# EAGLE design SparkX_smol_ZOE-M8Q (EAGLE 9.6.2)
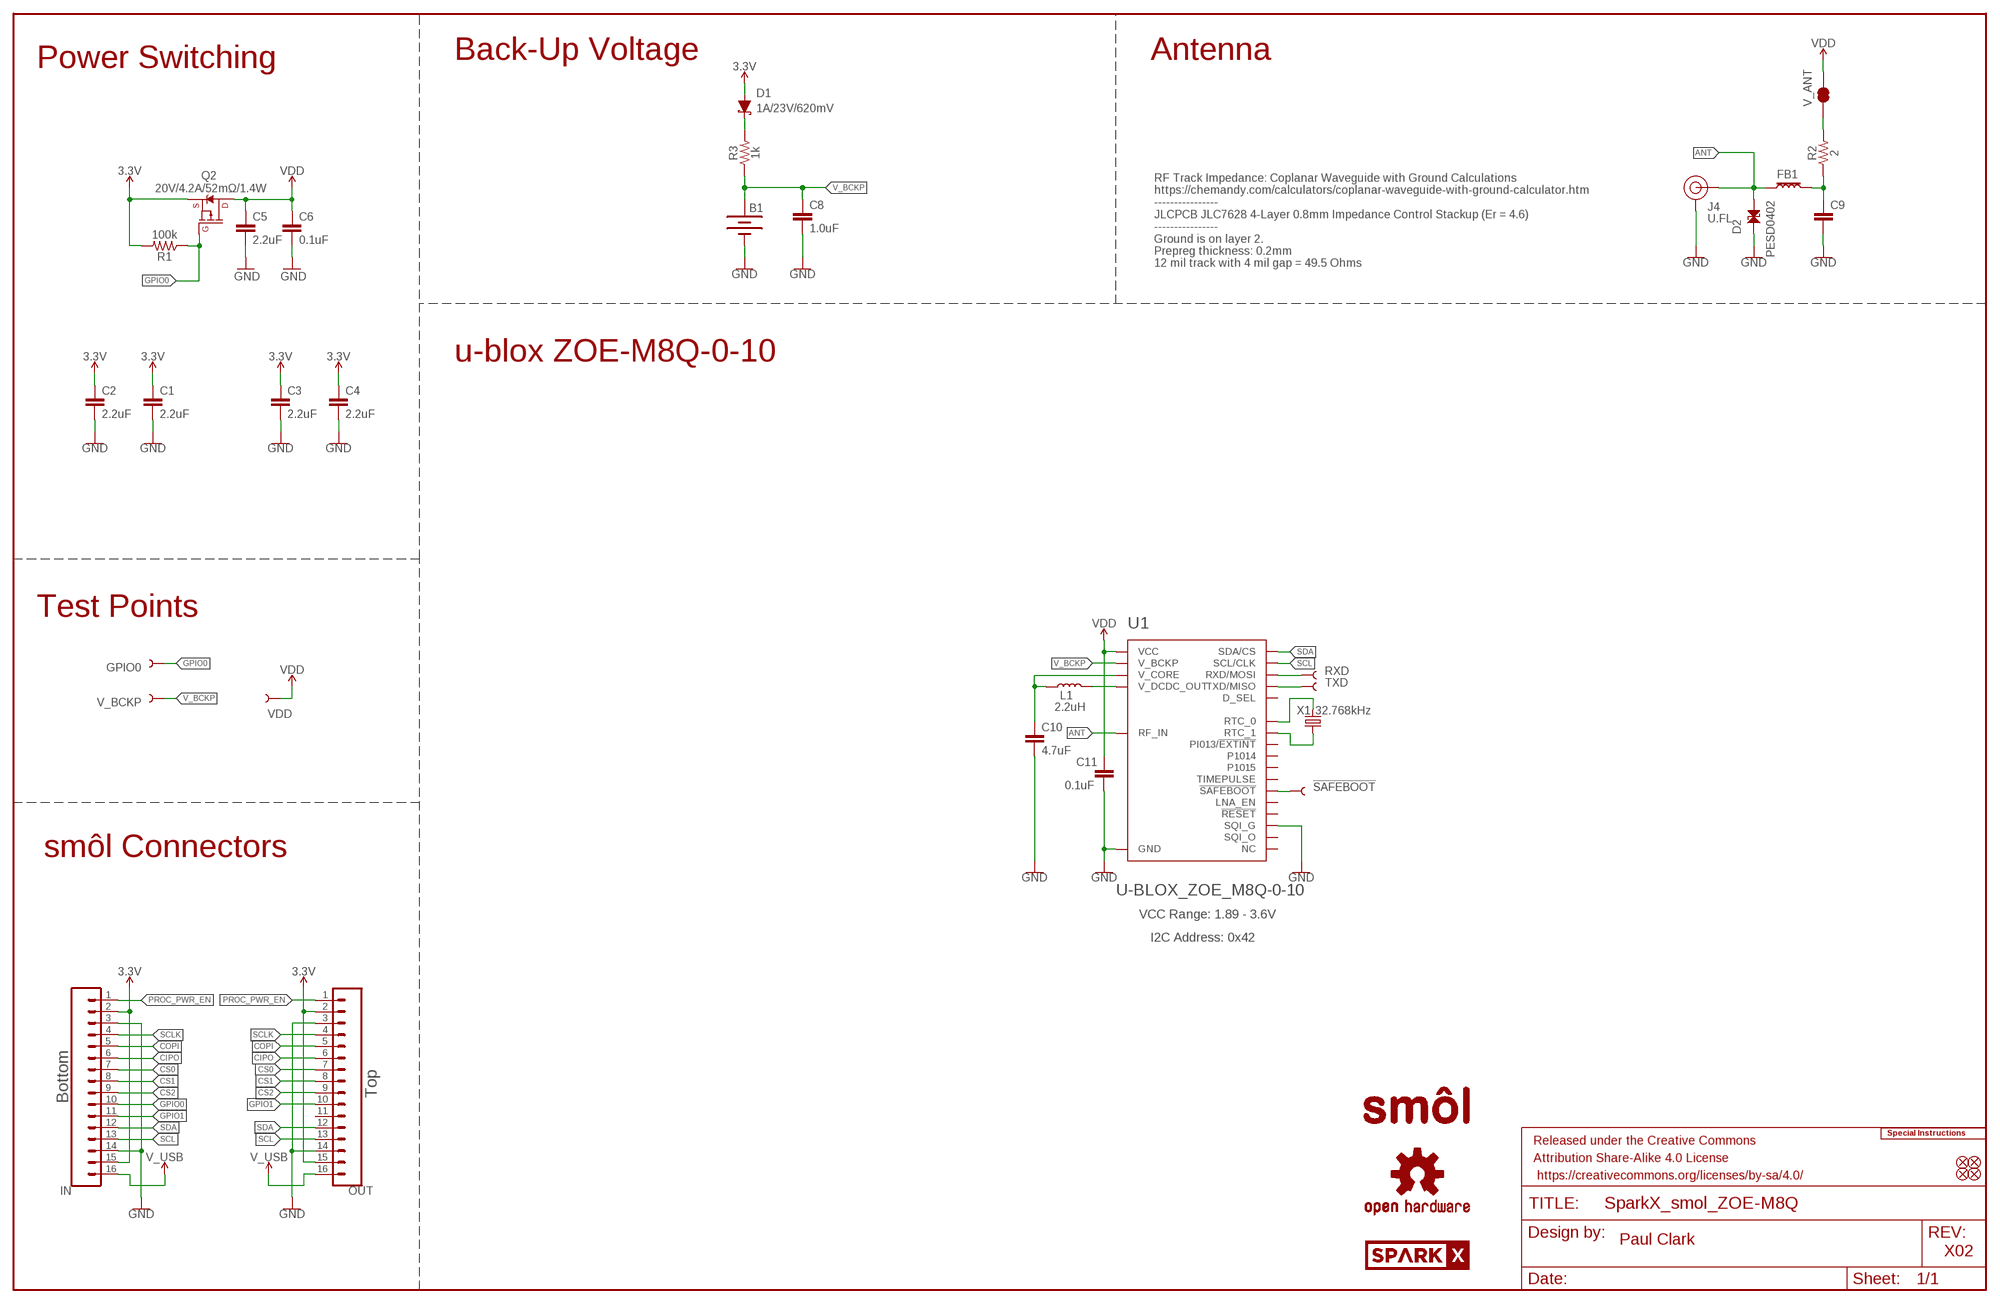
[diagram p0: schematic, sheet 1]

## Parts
!SAFEBOOT!  TEST-POINT3  [PAD.03X.03]
B1  6.8MM_COIN_CELL  ML414H_IV01E_BATTERY  [ML414H_IV01E]
C1  2.2uF  2.2UF-0402_TIGHT-10V-10%-X5R  [0402-TIGHT]
C2  2.2uF  2.2UF-0402_TIGHT-10V-10%-X5R  [0402-TIGHT]
C3  2.2uF  2.2UF-0402_TIGHT-10V-10%-X5R  [0402-TIGHT]
C4  2.2uF  2.2UF-0402_TIGHT-10V-10%-X5R  [0402-TIGHT]
C5  2.2uF  2.2UF-0402_TIGHT-10V-10%-X5R  [0402-TIGHT]
C6  0.1uF  0.1UF-0402T-10V-10%-X7R  [0402-TIGHT]
C8  1.0uF  1.0UF-0402T-16V-10%  [0402-TIGHT]
C9  47PF-0402_TIGHT-25V-5%-X7R  [0402-TIGHT]
C10  4.7uF  4.7UF-0402_TIGHT-6.3V-20%-X5R  [0402-TIGHT]
C11  0.1uF  0.1UF-0402T-6.3V-10%-X7R  [0402-TIGHT]
D1  1A/23V/620mV  DIODE-SCHOTTKY-BAT20J  [SOD-323]
D2  PESD0402  [0402]
FB1  FERRITE_BEAD-120_OHM-0402  [0402]
FD1  FIDUCIALUFIDUCIAL  [FIDUCIAL-MICRO]
FD2  FIDUCIALUFIDUCIAL  [FIDUCIAL-MICRO]
FD3  FIDUCIALUFIDUCIAL  [FIDUCIAL-MICRO]
FD4  FIDUCIALUFIDUCIAL  [FIDUCIAL-MICRO]
FRAME1  FRAME-LEDGER  [CREATIVE_COMMONS]
GPIO0  TEST-POINT3  [PAD.03X.03]
IN  CONN_16FPC_16_0.5MM  [FPC_16_0.5MM]
J4  U.FL  U.FL2PIN  [U.FL]
L1  2.2uH  2.2μH_SHIELDED_INDUCTOR  [0806]
LOGO1  SPECIAL_INSTRUCTIONS-ORDERING  [ORDERING_INSTRUCTIONS]
LOGO2  OSHW-LOGOMINI  [OSHW-LOGO-MINI]
LOGO3  OSHW-LOGOMINI  [OSHW-LOGO-MINI]
OUT  CONN_16FPC_16_0.5MM  [FPC_16_0.5MM]
Q2  20V/4.2A/52mΩ/1.4W  MOSFET_PCH-DMG2305UX-7  [SOT23-3]
R1  100k  100KOHM-0402T-1/16W-1%  [0402-TIGHT]
R2  2  2OHM-0402T-1/16W-1%  [0402-TIGHT]
R3  1k  1KOHM-0402T-1/16W-1%  [0402-TIGHT]
RXD  TEST-POINT3  [PAD.03X.03]
TXD  TEST-POINT3  [PAD.03X.03]
U1  U-BLOX_ZOE_M8Q-0-10  [UBLOX_ZOE_M8-0-10]
U$1  SPARKX-LOGO3  [SPARKX-SMALL]
U$3  SMOL_LOGOSMALL  [SMOL_SMALL]
U$4  SPARKX-LOGO3  [SPARKX-SMALL]
U$13  SMOL_LOGOSMALL  [SMOL_SMALL]
V_ANT  JUMPER-SMT_2_NC_TRACE_SILK  [SMT-JUMPER_2_NC_TRACE_SILK]
V_BCKP  TEST-POINT3  [PAD.03X.03]
VDD  TEST-POINT3  [PAD.03X.03]
X1  32.768kHz  CRYSTAL-32.768KHZSMD-3.2X1.5  [CRYSTAL-SMD-3.2X1.5MM]

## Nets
3.3V: C1.1 C2.1 C3.1 C4.1 D1.A IN.2 IN.15 OUT.2 OUT.15 Q2.2(S) R1.2
!SAFEBOOT!: !SAFEBOOT!.1 U1.34(!SAFEBOOT)
ANT: D2.2 FB1.1 J4.FEED(SIGNAL) U1.4(RF_IN)
CIPO: IN.6 OUT.6
COPI: IN.5 OUT.5
CS0: IN.7 OUT.7
CS1: IN.8 OUT.8
CS2: IN.9 OUT.9
GND: B1.- C1.2 C2.2 C3.2 C4.2 C5.2 C6.2 C8.2 C9.2 C10.2 C11.2 D2.1 IN.3 IN.14 J4.1(GND) J4.2(GND) OUT.3 OUT.14 U1.1(GND) U1.3(GND) U1.5(GND) U1.7(GND) U1.8(GND) U1.9(GND) U1.10(GND) U1.11(GND) U1.12(GND) U1.17(GND) U1.23(GND) U1.29(SQI_G) U1.31(SQI_G) U1.37(GND) U1.38(GND) U1.39(GND) U1.40(GND) U1.41(GND) U1.44(GND) U1.46(SQI_G) U1.47(SQI_G) U1.49(GND)
GPIO0: GPIO0.1 IN.10 Q2.1(G) R1.1
GPIO1: IN.11 OUT.10
N$4: R2.2 V_ANT.1
N$6: D1.C R3.2
N$22: L1.2 U1.26(V_DCDC_OUT)
N$23: C10.1 L1.1 U1.27(V_CORE)
N$27: U1.18(RTC_0) X1.P$2
N$32: U1.19(RTC_1) X1.P$1
N$34: C9.1 FB1.2 R2.1
PROC_PWR_EN: IN.1 OUT.1
RXD: RXD.1 U1.22(RXD/MOSI)
SCL: IN.13 OUT.13 U1.32(SCL/CLK)
SCLK: IN.4 OUT.4
SDA: IN.12 OUT.12 U1.2(SDA/CS)
TXD: TXD.1 U1.21(TXD/MISO)
V_BCKP: B1.+ C8.1 R3.1 U1.16(V_BCKP) V_BCKP.1
V_USB: IN.16 OUT.16
VDD: C5.1 C6.1 C11.1 Q2.3(D) U1.24(VCC) U1.25(VCC) V_ANT.2 VDD.1
Unconnected: OUT.11 U1.6(NC) U1.13(NC) U1.14(NC) U1.15(NC) U1.20(!RESET) U1.28(NC) U1.30(SQI_O) U1.33(TIMEPULSE) U1.35(LNA_EN) U1.36(P1015) U1.42(NC) U1.43(PI013/!EXTINT) U1.45(SQI_O) U1.48(D_SEL) U1.50(P1014) U1.51(NC)

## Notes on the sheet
- Power Switching | Back-Up Voltage | Antenna
- RF Track Impedance: Coplanar Waveguide with Ground Calculations
  https://chemandy.com/calculators/coplanar-waveguide-with-ground-calculator.htm
  ----------------
  JLCPCB JLC7628 4-Layer 0.8mm Impedance Control Stackup (Er = 4.6)
  ----------------
  Ground is on layer 2.
  Prepreg thickness: 0.2mm
  12 mil track with 4 mil gap = 49.5 Ohms
- u-blox ZOE-M8Q-0-10
- Test Points
- smôl Connectors
- VCC Range: 1.89 - 3.6V
- I2C Address: 0x42
- Top
- Bottom
- Paul Clark
- X02

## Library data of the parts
!SAFEBOOT! GPIO0 RXD TXD V_BCKP VDD = SparkFun-Connectors:TEST-POINT: SparkFun Test Points
B1 = SparkFun-Batteries:ML414H_IV01E_BATTERY: SEIKO ML414H-IV01E Reflowable Lithium Battery; PROD_ID: BATT-14267
C1-C5 = SparkFun-Capacitors:2.2UF: 2.2µF ceramic capacitors; PROD_ID: CAP-14232
C6 = SparkFun-Capacitors:0.1UF: 0.1µF ceramic capacitors; PROD_ID: CAP-15083
C8 = SparkFun-Capacitors:1.0UF: 1µF ceramic capacitors; PROD_ID: CAP-12417
C9 = SparkFun-Capacitors:47PF: 47pF ceramic capacitors; PROD_ID: CAP-15063
C10 = SparkFun-Capacitors:4.7UF: 4.7µF ceramic capacitors; PROD_ID: CAP-14240
C11 = SparkFun-Capacitors:0.1UF: 0.1µF ceramic capacitors; PROD_ID: CAP-14993
D1 = SparkFun-DiscreteSemi:DIODE-SCHOTTKY: Schottky diode; PROD_ID: DIO-11623
D2 = SparkFun-DiscreteSemi:PESD0402: ESD protection diode; DIGIKEY_PART: PESD0402-140CT-ND; MOUSE_PART: 650-PESD0402-140; PROD_ID: DIO-15359
FB1 = SparkFun-Coils:FERRITE_BEAD-120_OHM: Ferrite Bead (blocks, cores, rings, chokes, etc.); MFG_PART: BLM15HB121SN1D; PROD_ID: NDUC-14206
FD1-FD4 = SparkFun-Aesthetics:FIDUCIAL: Fiducial Alignment Points
FRAME1 = SparkFun-Aesthetics:FRAME-LEDGER: Schematic Frame - Ledger
IN OUT = SparkFun-Connectors:CONN_16: Multi connection point. Often used as Generic Header-pin footprint for 0.1 inch spaced/style header connections On any of the 0.1 inch spaced packages, you can populate with these: Break Away Headers - Straight (PRT-00116) Break Away Male Headers - Right Angle (PRT-00553) Female Headers (PRT-00115)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; PROD_ID: CONN-16066
J4 = SparkFun-Connectors:U.FL2PIN: SMD Antenna Connector - U.FL; PROD_ID: CONN-09193; SF_ID: WRL-09144
L1 = SparkFun-Coils:2.2μH_SHIELDED_INDUCTOR: Murata 2.2uH Inductor; PROD_ID: NDUC-14257
LOGO1 = SparkFun-Aesthetics:SPECIAL_INSTRUCTIONS: Special Ordering/Production Instructions Alert
LOGO2 LOGO3 = SparkFun-Aesthetics:OSHW-LOGO: Open-Source Hardware (OSHW) Logo
Q2 = SparkFun-DiscreteSemi:MOSFET_PCH: P-channel MOSFETs Voltage controlled devices that allow control of high current outputs. SparkFun Products: SparkFun ESP32 Thing SparkFun ESP8266 Thing SparkFun Pi Servo HAT V2 DMG2305UX-7 (20V/4.2A/SOT23-3); PROD_ID: TRANS-14388
R1 = SparkFun-Resistors:100KOHM: 100kΩ resistor; PROD_ID: RES-13495
R2 = SparkFun-Resistors:2OHM: 2 Ω resistor; PROD_ID: RES-15724
R3 = SparkFun-Resistors:1KOHM: 1kΩ resistor; PROD_ID: RES-14342
U1 = SparkFun-GPS:U-BLOX_ZOE_M8Q-0-10: UBLOX ZOE-M8Q-0-10 u-blox ZOE-M8 standard precision GNSS SiP (System in Package) modules feature the high performance u-blox M8 GNSS engine. ZOE-M8’s ultra-miniature form factor integrates a complete GNSS receiver including SAW filter, LNA and TCXO. Handles all GNSS systems and can simulatenously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; PROD_ID: IC-14251
U$1 U$4 = SparkX:SPARKX-LOGO
U$3 U$13 = SparkX:SMOL_LOGO
V_ANT = SparkFun-Jumpers:JUMPER-SMT_2_NC_TRACE: Normally closed trace jumper
X1 = SparkFun-Clocks:CRYSTAL-32.768KHZ: 32.768kHz Crystal; PROD_ID: XTAL-13062

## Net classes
1 Power: width 0.305 mm
2 3.3V: width 0.508 mm

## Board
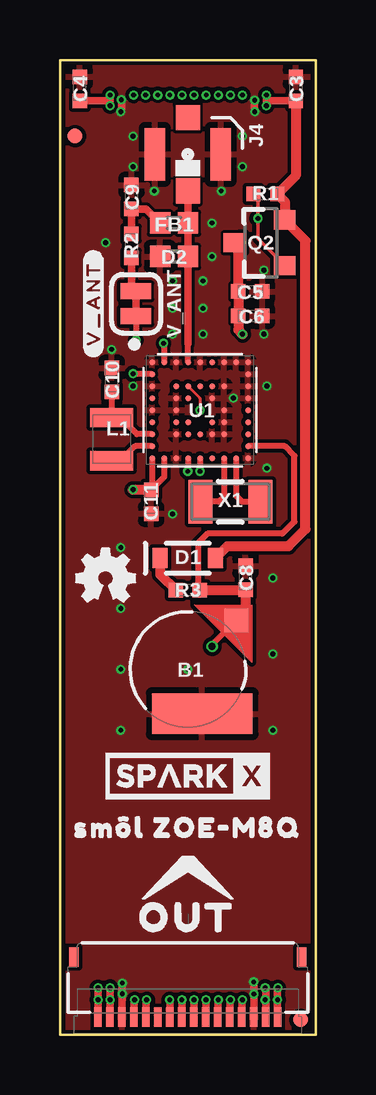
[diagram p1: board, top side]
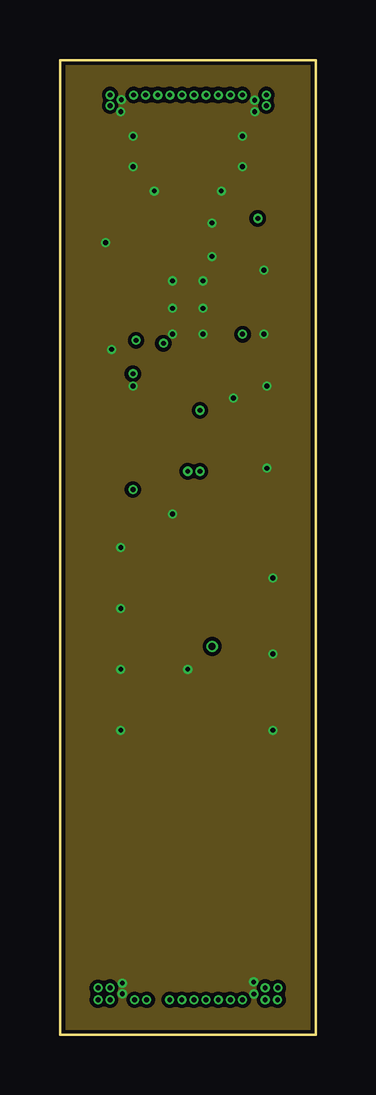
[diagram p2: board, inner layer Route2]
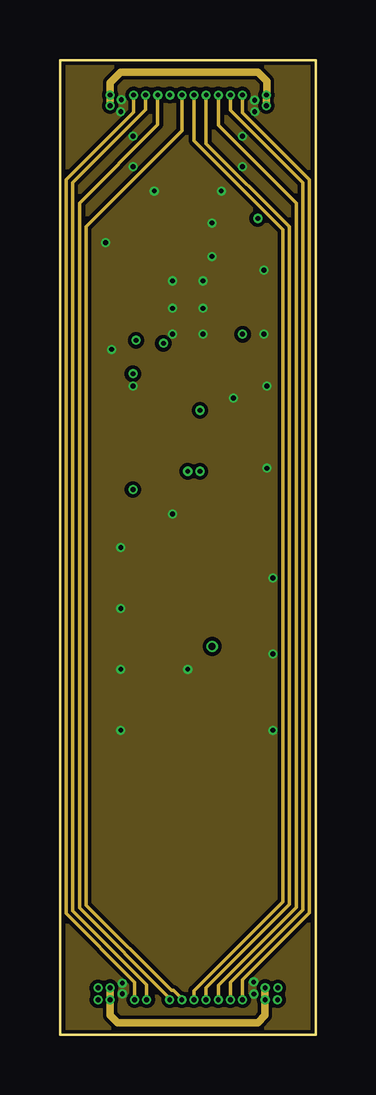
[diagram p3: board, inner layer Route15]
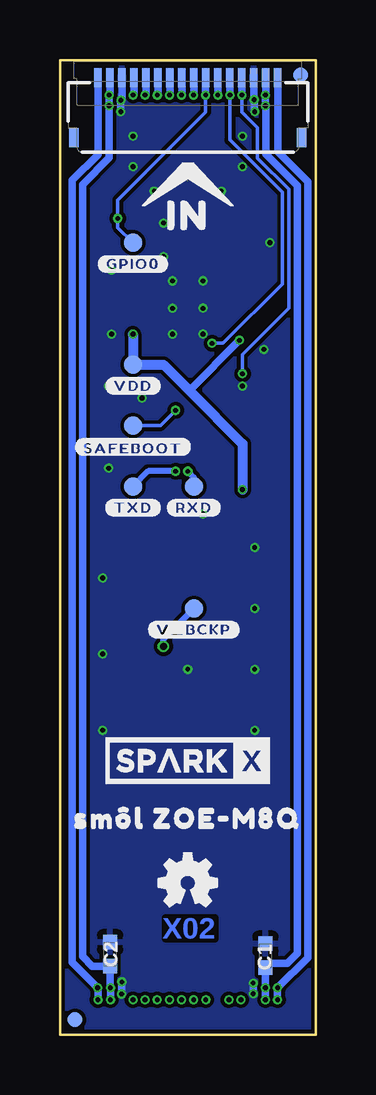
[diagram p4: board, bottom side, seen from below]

Size 10.67 x 40.64 mm. Coordinates in mm from the lower left corner, seen from the top.
Outline: 0,40.64 0,0 10.67,0 10.67,40.64 0,40.64
Copper layers (1+2*15+16): Top 0.035mm / dielectric 0.2mm / Route2 0.0175mm / dielectric 0.265mm / Route15 0.0175mm / dielectric 0.2mm / Bottom 0.035mm
Design rules "SparkFun-4_layer-Impedance_Control-JLCPCB-JLC7628": minimum track width 5mil, minimum drill 0.2mm, track to track 5mil, track to pad 5mil, pad to pad 5mil, via to via 5mil, smd to smd 0mil, copper to edge 5mil, drill to drill 5mil, minimum pad ring 3.5mil, minimum via ring 3.5mil, stop-mask expansion 2.5mil, vias tented up to drill 25mil, thermal gap 10mil

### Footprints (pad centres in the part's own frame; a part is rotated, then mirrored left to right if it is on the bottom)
PAD.03X.03 = smd 0.762 x 0.762: 1 0,0
ML414H_IV01E = smd 1 x 1: + 2.022,2.032 | smd 4.2 x 1.7: - 0.6,-1.85
0402-TIGHT = smd 0.6 x 0.6: 1 -0.5,0; 2 0.5,0
SOD-323 = smd 0.63 x 0.83: A 1.15,0; C -1.15,0
0402 = smd 0.85 x 0.9: 1 -0.58,0; 2 0.58,0
FIDUCIAL-MICRO = smd 0.635 x 0.635: 1 0,0
FPC_16_0.5MM = smd 0.3 x 0.8: 1 -3.75,1.35; 2 -3.25,1.35; 3 -2.75,1.35; 4 -2.25,1.35; 5 -1.75,1.35; 6 -1.25,1.35; 7 -0.75,1.35; 8 -0.25,1.35; 9 0.25,1.35; 10 0.75,1.35; 11 1.25,1.35; 12 1.75,1.35; 13 2.25,1.35; 14 2.75,1.35; 15 3.25,1.35; 16 3.75,1.35 | smd 0.4 x 0.8: MP1 -4.75,-1.15; MP2 4.75,-1.15
U.FL = smd 2.2 x 0.85: 1 0,1.375; 2 0,-1.375 | smd 1.05 x 1: FEED 1.525,0; NC -1.525,0
0806 = smd 0.8 x 1.8: 1 -0.9,0; 2 0.9,0
SOT23-3 = smd 0.8 x 0.9: 1 -0.95,-1; 2 0.95,-1; 3 0,1.1
UBLOX_ZOE_M8-0-10 = smd 0.25 x 0.25: 1 -1.996,2.004; 2 -1.496,2.004; 3 -0.996,2.004; 4 -0.496,2.004; 5 0.004,2.004; 6 0.504,2.004; 7 1.004,2.004; 8 1.504,2.004; 9 2.004,2.004; 10 2.004,1.504; 11 2.004,1.004; 12 2.004,0.504; 13 2.004,0.004; 14 2.004,-0.496; 15 2.004,-0.996; 16 2.004,-1.496; 17 2.004,-1.996; 18 1.504,-1.996; 19 1.004,-1.996; 20 0.504,-1.996; 21 0.004,-1.996; 22 -0.496,-1.996; 23 -0.996,-1.996; 24 -1.496,-1.996; 25 -1.996,-1.996; 26 -1.996,-1.496; 27 -1.996,-0.996; 28 -1.996,-0.496; 29 -1.996,0.004; 30 -1.996,0.504; 31 -1.996,1.004; 32 -1.996,1.504; 33 -0.996,1.004; 34 -0.496,1.004; 35 0.004,1.004; 36 0.504,1.004; 37 1.004,1.004; 38 1.004,0.004; 39 1.004,-0.496; 40 1.004,-0.996; 41 0.504,-0.996; 42 0.004,-0.996; 43 -0.496,-0.996; 44 -0.996,-0.996; 45 -0.996,-0.496; 46 -0.996,0.004; 47 -0.996,0.504; 48 -0.496,0.504; 49 0.504,0.504; 50 0.504,-0.496; 51 -0.496,-0.496
SMT-JUMPER_2_NC_TRACE_SILK = smd 0.66 x 1.27: 1 -0.521,0; 2 0.521,0
CRYSTAL-SMD-3.2X1.5MM = smd 1 x 1.8: P$1 -1.25,0; P$2 1.25,0

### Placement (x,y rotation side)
!SAFEBOOT!  7.62,25.4 0 bottom
B1  5.33,15.24 0 top
C1  2.1,3.3 90 bottom
C2  8.57,3.37 90 bottom
C3  9.84,39.43 90 top
C4  0.83,39.43 90 top
C5  7.94,30.99 0 top
C6  7.94,29.97 0 top
C8  7.75,19.05 90 top
C9  2.98,34.92 90 top
C10  2.16,27.3 90 top
C11  3.81,22.23 270 top
D1  5.33,19.88 0 top
D2  4.76,32.45 0 top
FB1  4.76,33.85 180 top
FD1  0.64,37.47 0 top
FD2  0.64,40.01 0 bottom
FD3  10.03,0.64 0 top
FD4  10.03,0.64 0 bottom
FRAME1  not placed on the board
GPIO0  7.62,33.02 0 bottom
IN  5.33,38.54 0 bottom
J4  5.33,36.7 270 top
L1  2.16,24.83 270 top
LOGO1  not placed on the board
LOGO2  1.91,19.05 0 top
LOGO3  5.33,6.35 0 bottom
OUT  5.33,2.1 180 top
Q2  8.38,33.02 90 top
R1  8.57,35.05 0 top
R2  2.98,32.89 270 top
R3  5.33,18.54 180 top
RXD  5.08,22.86 0 bottom
TXD  7.62,22.86 0 bottom
U1  5.84,26.04 0 top
U$1  5.33,10.79 0 top
U$2  [SM�L_ZOE#M8Q0]  5.33,9.02 0 bottom
U$3  5.33,6.79 0 top
U$4  5.33,11.43 0 bottom
U$5  [#V_ANT#0]  1.4,30.48 90 top
U$6  [#VDD#0]  7.62,27.05 0 bottom
U$7  [##SAFEBOOT##0]  7.62,24.51 0 bottom
U$8  [#TXD#0]  7.62,21.97 0 bottom
U$9  [#RXD#0]  5.08,21.97 0 bottom
U$10  [#GPIO0#0]  7.62,32.13 0 bottom
U$11  [#V_BCKP#0]  5.08,16.89 0 bottom
U$12  [SM�L_ZOE#M8Q0]  5.33,8.64 0 top
U$13  5.33,35.69 0 bottom
U$14  [OUT0]  5.33,4.89 0 top
U$15  [IN0]  5.33,34.16 0 bottom
V_ANT  3.17,30.48 270 top
V_BCKP  5.08,17.78 0 bottom
VDD  7.62,27.94 0 bottom
X1  7.11,22.23 0 top

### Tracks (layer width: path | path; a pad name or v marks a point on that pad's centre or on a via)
3.3V  (via drill 0.2)
  Top 0.305: OUT.2 8.58,1.95 v8.56,1.97 | v8.62,39.18 8.62,38.92 | 8.62,38.92 v8.62,38.73 | C3.1 8.62,38.93 8.62,38.92 | v2.1,39.18 2.1,38.92 | 2.1,38.92 v2.1,38.73 | C4.1 2.09,38.93 2.1,38.92 | OUT.15 2.08,1.45 v2.1,1.46 v2.09,1.46 v2.09,1.97
  Top 0.406: C3.1 9.84,35.82 R1.2 9.38,34.74 Q2.2 10.24,33.11 10.24,21.08 9.53,20.37 6.98,20.37 D1.A
  Route15 0.305: v2.09,1.97 v2.1,1.97 v2.1,1.46 2.1,0.83 2.41,0.51 8.26,0.51 8.56,0.81 v8.56,1.46 v8.56,1.97 | v2.1,38.73 v2.1,39.18 2.1,39.69 2.54,40.13 8.26,40.13 8.64,39.75 8.64,39.2 v8.62,39.18 v8.62,38.73
  Bottom 0.305: v8.56,1.46 v8.56,1.97 8.57,1.98 C2.1 9.33,2.87 9.73,3.27 9.73,35.45 8.62,36.56 v8.62,38.73 v8.62,39.18 8.58,39.21 IN.2 | v2.1,1.46 v2.1,1.97 v2.09,1.97 C1.1 1.91,2.98 1.17,2.98 0.76,3.39 0.76,35.39 2.07,36.7 2.07,38.67 2.1,38.7 v2.1,38.73 v2.1,39.18 2.08,39.19 IN.15
  Bottom 0.406: C2.1 8.58,2.86
!SAFEBOOT!  (via drill 0.2)
  Top 0.127: U1.34 5.84,26.54 v5.84,26.04
  Bottom 0.152: !SAFEBOOT!.1 6.48,25.4 v5.84,26.04
ANT
  Top 0.254: U1.4 5.35,28.82
  Top 0.305: FB1.1 | FB1.1 J4.FEED | FB1.1 D2.2 5.35,28.82
CIPO  (via drill 0.2)
  Top 0.305: v6.61,1.46 6.58,1.44 OUT.6
  Route15 0.152: v6.61,39.18 6.61,37.92 9.86,34.67 9.86,5.32 6.61,2.07 v6.61,1.46
  Bottom 0.305: IN.6 6.58,39.2 v6.61,39.18
COPI  (via drill 0.2)
  Top 0.305: v7.11,1.46 7.08,1.43 OUT.5
  Route15 0.152: v7.11,39.18 7.11,38.55 10.13,35.52 10.13,5.21 7.11,2.18 v7.11,1.46
  Bottom 0.305: IN.5 7.08,39.21 v7.11,39.18
CS0  (via drill 0.2)
  Top 0.305: OUT.7 6.08,1.45 v6.1,1.46
  Route15 0.152: v6.1,39.18 6.1,37.16 9.58,33.69 9.58,5.44 6.1,1.96 v6.1,1.46
  Bottom 0.305: IN.7 6.08,39.2 v6.1,39.18
CS1  (via drill 0.2)
  Top 0.305: OUT.8 v5.58,1.45 v5.59,1.46
  Route15 0.152: v5.6,39.18 5.6,37.27 9.3,33.57 9.3,5.55 5.59,1.85 v5.59,1.46
  Bottom 0.305: IN.8 5.58,39.19 v5.6,39.18
CS2  (via drill 0.2)
  Top 0.305: OUT.9 v5.08,1.46 v5.09,1.46
  Route15 0.152: v5.09,1.46 5.09,1.51 4.74,1.85 4.65,1.85 1.09,5.41 1.09,33.69 5.09,37.68 v5.09,39.18
  Bottom 0.305: IN.9 v5.08,39.19 v5.09,39.18
GND  (via drill 0.2)
  Top 0.305: v8.12,38.96 v8.12,38.48 v8.13,38.48 | v2.56,38.99 2.56,38.51 v2.54,38.48 | OUT.14 2.58,1.7 v2.6,1.71 v2.6,2.16 | OUT.3 8.08,1.26 8.09,1.27 v8.09,1.7 v8.08,1.71 v8.08,2.21
  Bottom 0.305: IN.3 8.08,39 v8.12,38.96 v8.13,38.95 v8.13,38.48 | IN.14 2.58,39.01 v2.56,38.99 2.56,38.51 v2.54,38.48 | v2.6,1.71 v2.6,2.16 | v8.09,1.7 8.09,2.2 v8.08,2.21
  other vias: 7.62,37.47 7.62,36.2 3.05,36.2 3.05,37.47 3.94,35.18 6.73,35.18 8.51,31.88 8.51,29.21 6.35,33.85 5.97,31.43 5.97,29.21 5.97,30.29 4.7,29.21 4.7,30.29 4.7,31.43 2.16,28.57 8.89,19.05 3.05,27.05 8.64,27.05 8.64,23.62 4.7,21.72 1.91,33.02 2.54,17.78 2.54,20.32 5.33,15.24 7.24,26.54 2.54,15.24 2.54,12.7 8.89,12.7 8.89,15.88 6.35,32.45
  pour Top (isolate 0.152, rank 3): 0,40.64 10.67,40.64 10.67,0 0,0
  pour Route2 (isolate 0.152, rank 2): 0,40.64 10.67,40.64 10.67,0 0,0
  pour Route15 (isolate 0.152, rank 2): 0,40.64 10.67,40.64 10.67,0 0,0
  pour Bottom (isolate 0.152, rank 2): 0,40.64 10.67,40.64 10.67,0 0,0
  pour Top (isolate 0.102): 3.3,39.12 7.37,39.12 7.37,27.43 3.3,27.43
GPIO0  (via drill 0.2)
  Top 0.152: R1.1 8.26,34.87 8.26,34.29 v8.26,34.04 8.26,33.2 Q2.1
  Bottom 0.152: v4.59,39.18 4.59,38.47 8.26,34.8 v8.26,34.04 8.26,33.66 GPIO0.1
  Bottom 0.305: IN.10 v4.59,39.18
GPIO1  (via drill 0.2)
  Top 0.305: OUT.10 v4.58,1.46
  Route15 0.152: v4.08,39.18 4.08,37.95 0.81,34.67 0.81,5.29 4.58,1.53 v4.58,1.46
  Bottom 0.305: IN.11 v4.08,39.18
N$4
  Top 0.305: V_ANT.1 2.98,31.19 R2.2
N$6
  Top 0.406: D1.C 4.18,19.19 R3.2
N$22
  Top 0.254: U1.26 3.14,24.54 2.53,23.93 L1.2
N$23
  Top 0.254: C10.1 L1.1 2.53,25.73 3.22,25.04 U1.27
N$27
  Top 0.254: U1.18 7.35,22.48 7.6,22.23 X1.P$2
N$32
  Top 0.254: U1.19 6.85,22.45 6.62,22.23 X1.P$1
N$34
  Top 0.305: FB1.2 3.6,34.42 C9.1 R2.1
PROC_PWR_EN  (via drill 0.2)
  Top 0.305: OUT.1 v9.08,1.46 9.08,1.95 v9.09,1.96
  Bottom 0.305: v9.08,1.46 9.08,1.95 v9.09,1.96 10.16,3.02 10.16,35.62 9.08,36.7 IN.1
RXD  (via drill 0.2)
  Top 0.254: U1.22 5.35,23.51 v5.33,23.5
  Bottom 0.254: v5.33,23.5 5.08,23.24 RXD.1
SCL  (via drill 0.2)
  Top 0.254: U1.32 3.07,27.54 v3.05,27.56
  Top 0.305: OUT.13 3.08,1.43 v3.12,1.46
  Route15 0.152: v3.07,39.18 3.07,38.46 0.25,35.64 0.25,5.06 3.12,2.2 v3.12,1.46
  Bottom 0.152: v3.05,27.56 3.05,28.36 1.12,30.29 1.12,35.25 2.43,36.56 2.43,37.81 3.07,38.46 v3.07,39.18
  Bottom 0.305: IN.13 v3.07,39.18
SCLK  (via drill 0.2)
  Top 0.305: v7.62,1.46 7.58,1.43 OUT.4
  Route15 0.152: v7.62,1.46 7.62,2.3 10.41,5.09 10.41,35.64 7.62,38.44 v7.62,39.18
  Bottom 0.305: v7.62,39.18 7.58,39.21 IN.4
SDA  (via drill 0.2)
  Top 0.254: v4.32,28.83 4.35,28.8 U1.2
  Top 0.305: OUT.12 3.58,1.43 v3.62,1.46
  Route15 0.152: v3.62,1.46 3.62,2.09 0.53,5.18 0.53,35.52 3.58,38.57 v3.58,39.18
  Bottom 0.152: v3.58,39.18 3.58,37.31 1.4,35.13 1.4,31.29 3.86,28.83 v4.32,28.83
  Bottom 0.305: IN.12 v3.58,39.19 v3.58,39.18
TXD  (via drill 0.2)
  Top 0.254: U1.21 v5.85,23.5 v5.84,23.5
  Bottom 0.254: v5.84,23.5 6.99,23.5 TXD.1
V_BCKP  (via drill 0.3)
  Top 0.254: U1.16 9.38,24.54 9.79,24.13 9.79,21.4 9.28,20.89 6.16,20.89 5.77,20.5 5.77,18.61 R3.1 | B1.+ 6.35,16.27 v6.35,16.19
  Top 0.406: R3.1 C8.1 7.75,17.66 B1.+
  Bottom 0.254: v6.35,16.19 6.35,16.51 V_BCKP.1
V_USB  (via drill 0.2)
  Top 0.305: OUT.16 v1.59,1.46 v1.59,1.96
  Bottom 0.305: IN.16 1.58,36.83 0.33,35.57 0.33,3.21 v1.59,1.96 v1.59,1.46
VDD  (via drill 0.2)
  Top 0.254: U1.25 3.85,22.76 | 3.85,22.76 C11.1 | U1.24 4.35,23.26 3.85,22.76 | V_ANT.2 v3.17,28.96
  Top 0.406: v7.62,29.21 7.44,29.39 C6.1 C5.1 7.44,32.86 Q2.3 | v3.05,22.73 C11.1 3.85,22.76
  Bottom 0.305: v3.17,28.96 5.27,26.86
  Bottom 0.406: v7.62,29.21 VDD.1 6.35,27.94 5.27,26.86 3.05,24.64 v3.05,22.73

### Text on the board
Bottom: X02
Measures: Dimensions in Inches
tDocu: JLCPCB JLC7628 4-Layer 0.8mm Impedance Control / 4-Layer Board / 0.8mm Thickness / 1oz Copper (Outer layers) / ENIG Finish | Paul Clark

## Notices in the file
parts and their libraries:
SparkFun-Aesthetics: Licensing: Creative Commons ShareAlike 4.0 International - https://creativecommons.org/licenses/by-sa/4.0
SparkFun-Aesthetics: Released under the Creative Commons Attribution Share-Alike 4.0 License
SparkFun-Aesthetics: https://creativecommons.org/licenses/by-sa/4.0
